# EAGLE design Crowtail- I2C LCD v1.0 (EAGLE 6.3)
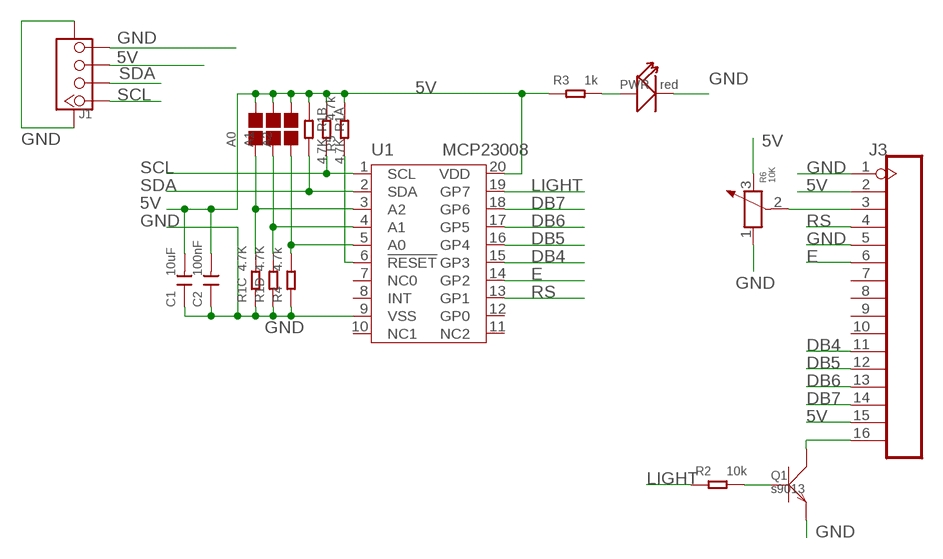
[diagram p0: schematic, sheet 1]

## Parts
A0  PAD-JUMPER-2P  [2P-SMD-1.78X1.27]
A1  PAD-JUMPER-2P  [2P-SMD-1.78X1.27]
A2  PAD-JUMPER-2P  [2P-SMD-1.78X1.27]
C1  10uF  C-0805  [0805]
C2  100nF  C-0603  [0603]
J1  TWIG-4P-2.0-SMD-FEMALE-REINFORCE'90D'  [4P-SMD-2.0-90D]
J3  HEADER-16P-2.54  [16P-2.54]
PWR  red  LED'0603'  [LED-0603]
Q1  s9013  TRANSISTOR-NPN-SOT23  [SOT23]
R1  4.7K  R-4R-1206  [1206-8-3.3X2.4]
R2  10k  R-0603  [0603]
R3  1k  R-0603  [0603]
R4  4.7k  R-0603  [0603]
R5  4.7k  R-0603  [0603]
R6  10K  R-POTENTIOMETER-SMD  [3P-SMD-SQUA-3.6X3.3]
U1  MCP23008  [SSOP20]

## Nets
5V: A0.1 A1.1 A2.1 C1.2 C2.2 J1.3 J3.2 J3.15 R1.1 R1.2 R3.1 R5.2 R6.3 U1.20(VDD)
DB4: J3.11 U1.15(GP3)
DB5: J3.12 U1.16(GP4)
DB6: J3.13 U1.17(GP5)
DB7: J3.14 U1.18(GP6)
E: J3.6 U1.14(GP2)
GND: C1.1 C2.1 J1.4 J1.SS1 J1.SS2 J3.1 J3.5 PWR.- Q1.2(E) R1.3 R1.4 R4.1 R6.1 U1.9(VSS)
LIGHT: R2.1 U1.19(GP7)
N$2: Q1.1(B) R2.2
N$3: A0.2 R1.6 U1.3(A2)
N$4: A1.2 R1.5 U1.4(A1)
N$5: A2.2 R4.2 U1.5(A0)
N$6: R5.1 U1.6(!RESET)
N$7: J3.3 R6.2
N$8: PWR.+ R3.2
N$20: J3.16 Q1.3(C)
RS: J3.4 U1.13(GP1)
SCL: J1.1 R1.8 U1.1(SCL)
SDA: J1.2 R1.7 U1.2(SDA)
Unconnected: J3.7 J3.8 J3.9 J3.10 U1.7(NC0) U1.8(INT) U1.10(NC1) U1.11(NC2) U1.12(GP0)

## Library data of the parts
A0 A1 A2 = Discrete:PAD-JUMPER-2P; PARTNO: DNP
C1 C2 = Discrete:C*: Ceramic Capacitors
J1 = Connector:TWIG-4P-2.0-SMD-FEMALE-REINFORCE
J3 = Connector:HEADER-16P
PWR = Discrete:LED*
Q1 = Discrete:TRANSISTOR-NPN*: NPN audion
R1 = Discrete:R-4R*: Resistor Array
R2-R5 = Discrete:R*
R6 = Discrete:R-POTENTIOMETER*: Potentiometer
U1 = IC:MCP23008

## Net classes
1 power: width 0.61 mm, drill 0.406 mm, clearance 0.203 mm
2 gnd: width 0.305 mm, drill 0.559 mm, clearance 0.254 mm
3 usbvcc: width 0.508 mm, drill 0.61 mm, clearance 0.254 mm

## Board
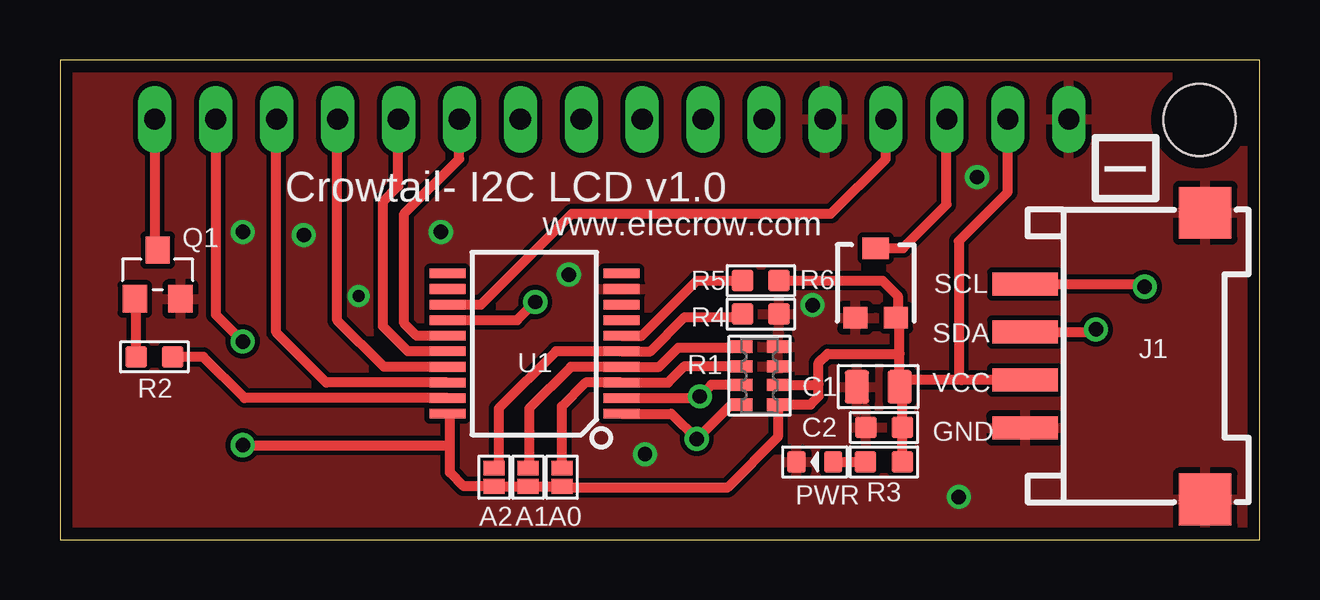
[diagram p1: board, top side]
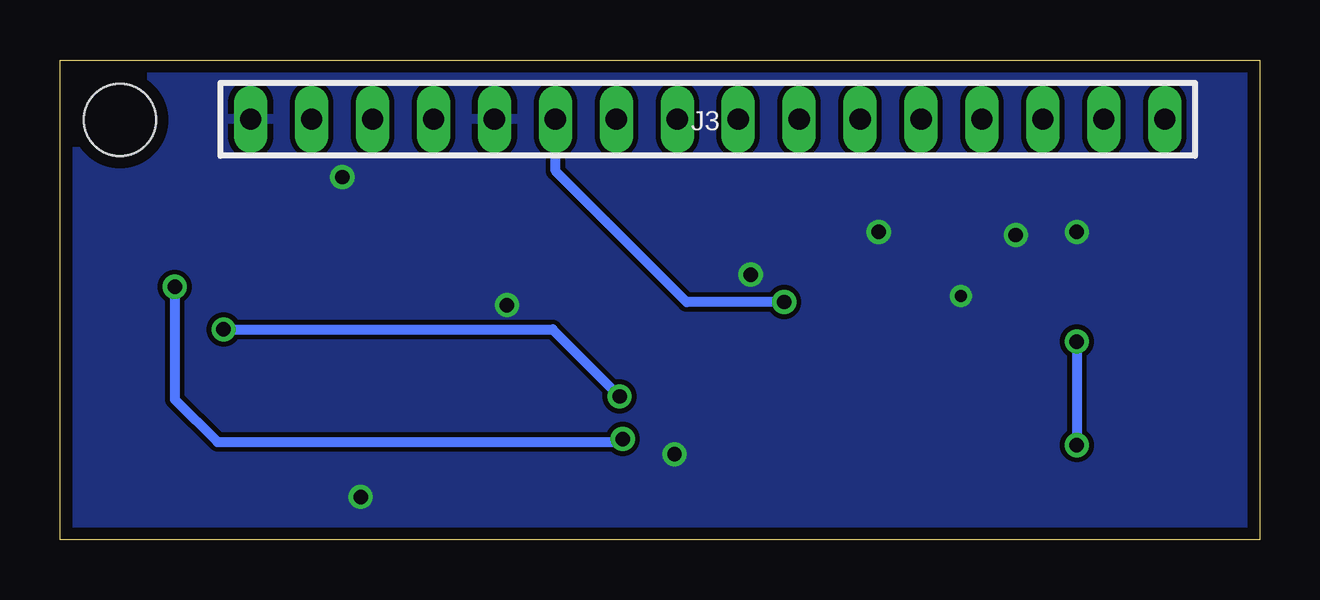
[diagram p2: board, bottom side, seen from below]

Size 50 x 20 mm. Coordinates in mm from the lower left corner, seen from the top.
Outline: 50,20 0,20 0,0 50,0 50,20
Copper layers (1*16): Top 0.035mm / dielectric 1.5mm / Bottom 0.035mm
Design rules "default *": minimum track width 10mil, minimum drill 20mil, track to track 8mil, track to pad 8mil, pad to pad 8mil, via to via 8mil, smd to smd 8mil, copper to edge 20mil, drill to drill 8mil, minimum pad ring 10mil, minimum via ring 8mil, stop-mask expansion 2mil, vias tented up to drill 100mil, thermal gap 10mil
Holes 3 mm at 47.5,17.5

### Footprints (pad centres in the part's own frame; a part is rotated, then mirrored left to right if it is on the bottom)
2P-SMD-1.78X1.27 = smd 0.889 x 0.61: 1 0,0.381; 2 0,-0.381
0805 = smd 1.016 x 1.397: 1 -0.889,0; 2 0.889,0
0603 = smd 0.889 x 0.889: 1 -0.762,0; 2 0.762,0
4P-SMD-2.0-90D = smd 0.965 x 2.74: 1 -3,-0.1; 2 -1,-0.1; 3 1,-0.1; 4 3,-0.1 | smd 2.159 x 2.184: SS1 -5.974,7.4; SS2 5.974,7.4
16P-2.54 = drill 0.889 long: 1 -19.05,0; 2 -16.51,0; 3 -13.97,0; 4 -11.43,0; 5 -8.89,0; 6 -6.35,0; 7 -3.81,0; 8 -1.27,0; 9 1.27,0; 10 3.81,0; 11 6.35,0; 12 8.89,0; 13 11.43,0; 14 13.97,0; 15 16.51,0; 16 19.05,0
LED-0603 = smd 0.762 x 0.889: + -0.762,0; - 0.762,0
SOT23 = smd 1.016 x 1.143: 1 -0.95,-1.016; 2 0.95,-1.016; 3 0,1.016
1206-8-3.3X2.4 = smd 0.508 x 0.914: 1 -1.206,-0.762; 2 -0.381,-0.762; 3 0.381,-0.762; 4 1.206,-0.762; 5 1.206,0.762; 6 0.381,0.762; 7 -0.381,0.762; 8 -1.206,0.762
3P-SMD-SQUA-3.6X3.3 = smd 1 x 0.9: 1 -0.85,-1.45; 3 0.85,-1.45 | smd 1.1 x 0.9: 2 0,1.45
SSOP20 = smd 0.4 x 1.5: 1 -2.925,-3.625; 2 -2.275,-3.625; 3 -1.625,-3.625; 4 -0.975,-3.625; 5 -0.325,-3.625; 6 0.325,-3.625; 7 0.975,-3.625; 8 1.625,-3.625; 9 2.275,-3.625; 10 2.925,-3.625; 11 2.925,3.625; 12 2.275,3.625; 13 1.625,3.625; 14 0.975,3.625; 15 0.325,3.625; 16 -0.325,3.625; 17 -0.975,3.625; 18 -1.625,3.625; 19 -2.275,3.625; 20 -2.925,3.625

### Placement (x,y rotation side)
A0  20.93,2.6 180 top
A1  19.51,2.6 180 top
A2  18.1,2.6 180 top
C1  34.11,6.37 0 top
C2  34.35,4.67 0 top
J1  40.33,7.65 270 top
J3  23,17.53 0 bottom
PWR  31.46,3.23 180 top
Q1  4.07,11.06 0 top
R1  29.16,6.83 90 top
R2  3.94,7.62 180 top
R3  34.34,3.23 180 top
R4  29.21,9.4 180 top
R5  29.21,10.79 0 top
R6  34,10.7 0 top
U1  19.77,8.17 90 top

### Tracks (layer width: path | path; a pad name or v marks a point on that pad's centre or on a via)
5V  (via drill 0.6)
  Top 0.406: R3.1 C2.2 35.11,6.26 C1.2 | C1.2 35,7.75 | 35,7.75 35,9.1 R6.3 34.92,9.32 34.92,10.16 34.29,10.79 R5.2 | J1.3 37.59,6.65 | 37.59,6.65 35.28,6.65 C1.2 | 37.59,6.65 37.47,6.78 37.47,12.45 39.51,14.49 J3.2 | 16.26,3.94 16.26,2.79 16.83,2.22 A2.1 A1.1 A0.1 20.99,2.16 27.81,2.16 29.93,4.27 R1.1 31.28,5.63 31.62,5.97 31.62,6.48 | 16.26,3.94 16.26,5.14 U1.20 | J3.15 6.49,9.38 v7.62,8.26 | v7.62,3.94 16.26,3.94 | 35,7.75 32,7.75 31.62,7.37 31.62,6.48 | R1.2 31.6,6.45 31.62,6.48
  Bottom 0.406: v7.62,8.26 v7.62,3.94
DB4
  Top 0.406: U1.15 14.87,8.5 14.35,9.02 14.35,13.59 16.64,15.88 16.64,17.52 J3.11
DB5
  Top 0.406: U1.16 14.5,7.85 13.46,8.89 13.46,14.1 14.1,14.73 14.1,17.52 J3.12
DB6
  Top 0.406: U1.17 13.5,7.2 11.56,9.14 11.56,17.52 J3.13
DB7
  Top 0.406: U1.18 11.1,6.55 9.02,8.64 9.02,17.52 J3.14
E  (via drill 0.6)
  Top 0.406: U1.14 19.05,9.15 v19.81,9.91
  Bottom 0.406: v19.81,9.91 23.88,9.91 29.34,15.37 29.34,17.52 J3.6
GND  (via drill 0.51, 0.6)
  other vias: 37.47,1.78 15.88,12.83 31.37,9.78 24.38,3.56 21.21,11.05 10.16,12.7 7.62,12.83 12.45,10.16 38.23,15.11
  pour Top: -1.82,20.22 51.91,20.19 51.91,-0.13 -1.82,-0.1
  pour Bottom: -2,19.9 51.78,20.19 51.78,-0.13 -2,-0.1
LIGHT
  Top 0.406: U1.19 7.69,5.9 5.97,7.62 R2.1
N$2
  Top 0.406: R2.2 3.17,9.99 Q1.1
N$3
  Top 0.406: R1.6 28.38,7.24 26.04,7.24 25.34,6.55 U1.3 21.92,6.55 20.93,5.56 A0.2
N$4
  Top 0.406: R1.5 28.36,8 25.78,8 24.98,7.2 U1.4 21.3,7.2 19.56,5.46 19.56,3.03 A1.2
N$5
  Top 0.406: R4.2 28.32,9.27 26.04,9.27 24.61,7.85 U1.5 20.68,7.85 18.29,5.46 18.29,3.17 A2.2
N$6
  Top 0.406: U1.6 24.25,8.5 26.54,10.79 R5.1
N$7
  Top 0.406: R6.2 35.14,12.15 36.96,13.97 36.96,17.52 J3.3
N$8
  Top 0.406: PWR.+ R3.2
N$20
  Top 0.406: J3.16 3.95,12.19 Q1.3
RS
  Top 0.406: U1.13 17.55,9.8 21.34,13.59 32.13,13.59 34.42,15.88 34.42,17.52 J3.4
SCL  (via drill 0.6)
  Top 0.406: U1.1 25.48,5.25 v26.54,4.19 27.98,5.63 R1.8 | J1.1 45.1,10.65 v45.21,10.54
  Bottom 0.406: v45.21,10.54 45.21,5.84 43.43,4.06 26.67,4.06 v26.54,4.19
SDA  (via drill 0.6)
  Top 0.406: U1.2 26.6,5.9 v26.67,5.97 27.16,6.45 R1.7 | J1.2 43.07,8.65 v43.18,8.76
  Bottom 0.406: v43.18,8.76 29.46,8.76 v26.67,5.97

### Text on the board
tPlace: I | Crowtail- I2C LCD v1.0 | www.elecrow.com | SCL | SDA | VCC | GND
